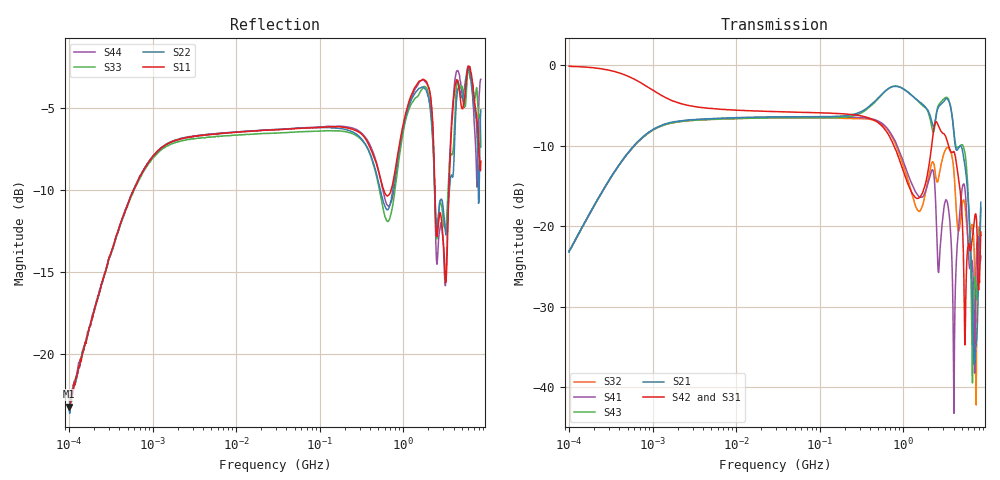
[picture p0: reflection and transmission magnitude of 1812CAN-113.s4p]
# Hz S dB R 50
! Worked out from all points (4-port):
!   801 points, 100 kHz to 8.5 GHz, reference 50 ohm
!   strongest paths, dB at 100 kHz, 1.721 MHz, 29.51 MHz, 502.3 MHz, 8.5 GHz:
!     S42: -0.1, -4.4, -5.8, -7.1, -20.7
!     S31: -0.1, -4.5, -5.8, -7.3, -24.0
!     S21: -23.2, -7.1, -6.4, -4.1, -17.0
!     S43: -23.1, -7.1, -6.5, -4.2, -17.7
!     S41: -23.2, -7.1, -6.4, -6.9, -23.7
!     S32: -23.1, -7.2, -6.6, -7.0, -21.2
!   lowest |S11| = -23.2 dB at 100 kHz (marker M1), VSWR 1.15, Z = 50.9 + j6.93 ohm
!   |S11| at or under -10 dB: start of sweep to 586.9 kHz; 586 MHz to 713.3 MHz (127.2 MHz wide, 19.6 % of centre); 2.392 GHz to 3.515 GHz (1.123 GHz wide, 38 % of centre)
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100000  -23.20 78.4  -23.16 81.6  -0.12 -3.9  -23.15 -99.4
        -23.21 81.6  -23.37 75.2  -23.10 -98.6  -0.14 -4.0
        -0.14 -3.8  -23.12 -98.8  -22.60 81.9  -23.09 81.1
        -23.19 -98.5  -0.11 -4.0  -23.05 80.3  -22.61 80.9
1952074  -6.92 18.4  -6.97 18.4  -4.67 -14.2  -7.00 -161.9
         -6.98 18.5  -6.90 18.3  -7.03 -162.0  -4.60 -14.1
         -4.66 -14.2  -7.06 -161.8  -7.06 18.4  -7.04 18.5
         -7.00 -161.9  -4.61 -14.2  -7.04 18.4  -6.92 18.3
1.665909e9  -3.27 61.2  -4.76 -23.4  -16.31 159.1  -16.41 35.3
            -4.75 -23.4  -3.71 60.9  -17.71 49.0  -16.03 157.2
            -16.31 159.3  -17.69 49.0  -3.85 62.0  -4.91 -22.1
            -16.40 35.2  -16.04 157.4  -4.90 -22.1  -3.28 61.8
4.048099e9  -4.24 -127.5  -8.59 -68.0  -10.80 -15.1  -43.33 13.6
            -8.57 -68.1  -8.14 -125.5  -13.31 -123.7  -10.76 -15.6
            -10.75 -15.1  -13.32 -123.9  -6.81 -130.7  -8.32 -60.6
            -43.26 16.4  -10.72 -15.6  -8.31 -60.5  -3.84 -128.7
4.713137e9  -3.94 -112.3  -10.10 -56.5  -15.18 -56.0  -18.78 42.4
            -10.10 -56.5  -3.84 -105.3  -20.23 105.8  -14.96 -54.1
            -15.16 -56.1  -20.23 105.8  -3.62 -107.9  -10.11 -47.8
            -18.82 42.6  -14.92 -54.1  -10.11 -47.6  -2.97 -114.9
7.256907e9  -4.83 29.1  -36.64 99.6  -17.84 0.9  -32.87 121.1
            -36.48 99.0  -5.35 22.5  -29.70 -68.1  -18.58 5.6
            -17.85 0.7  -29.77 -68.2  -4.35 35.9  -26.38 7.1
            -32.88 122.0  -18.56 5.7  -26.30 8.3  -6.78 17.6
8.5e9  -8.23 132.0  -17.04 96.8  -24.00 39.8  -23.76 51.4
       -17.01 96.7  -5.09 125.7  -21.14 41.0  -20.72 10.9
       -23.97 39.4  -21.15 40.3  -7.35 116.6  -17.68 74.6
       -23.72 51.3  -20.73 10.6  -17.70 74.9  -3.21 126.1
